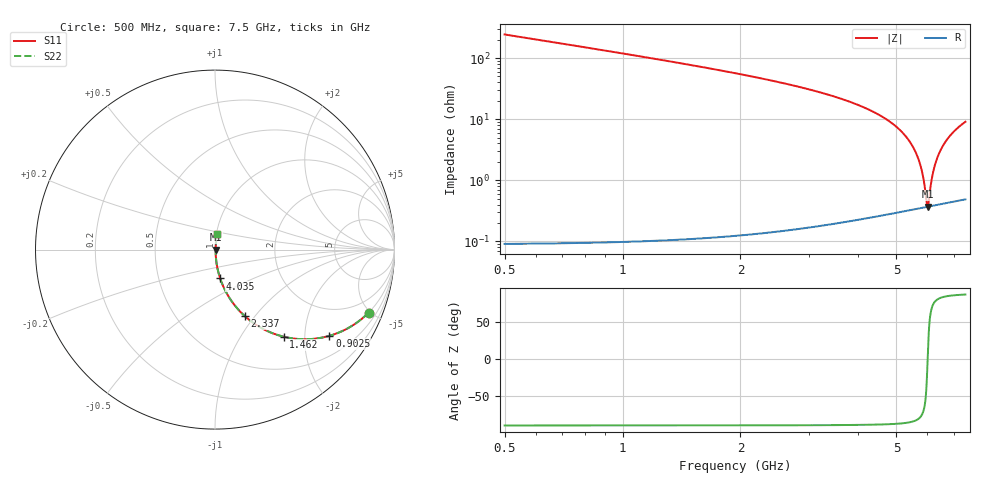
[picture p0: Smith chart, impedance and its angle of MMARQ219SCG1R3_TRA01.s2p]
! MMARQ219SCG1R3_TRA01  S-PARAMETER MODEL  ( General Type )
! Model Generated by TAIYO YUDEN Corporation (http://www.ty-top.com)
! Version 1.0
! TAIYO YUDEN Control No. 180601
! Copyright(c) 2018 TAIYO YUDEN CO.,LTD. All Rights Reserved.
! Product Description (link to TY-COMPAS)
! https://ds.yuden.co.jp/TYCOMPAS/or/detail?pn=MMARQ219SCG1R3BTRA01&u=M
! Products Name : Multilayer Ceramic Capacitors
! Characteristics :
!  Capacitance : 1.3 pF , Rated Voltage : 250V , TCC : CG / C0G
!  Case Size : 2.0 x 1.25 / 0.079 x 0.049 [mm/inch] , Thickness : 0.85 / 0.033 [mm/inch]
!  (Conditions: Temperature = 25 degC , DC Bias Current/Voltage = 0A / 0V)
! External Node Assignments :
!  1  o---| |---o  2
! GND o---------o GND
! Frequency Range : 500MHz  -  7500MHz  [ 401 STEP ]
# MHz S RI R 50
! Freq[MHz].  S11 Real  S11 Imag  S21 Real  S21 Imag  S12 Real  S12 Imag  S22 Real  S22 Imag
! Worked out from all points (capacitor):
!   401 points, 500 MHz to 7.5 GHz, reference 50 ohm
!   read as one part in series: C = 1.3 pF near 535 MHz
!   lowest |Z| = 370 mohm at 6.013 GHz (marker M1)
!   series resonance near 6.008 GHz, so ESL is about 540 pH
!   S11 on the Smith chart (normalised r, x): 500 MHz: 1.00, -4.86; 902.5 MHz: 1.00, -2.65; 1.462 GHz: 1.00, -1.57; 2.337 GHz: 1.00, -0.89; 4.035 GHz: 1.00, -0.33; 7.5 GHz: 1.01, +0.18
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500  0.8553 -0.3516  0.1447 0.3516  0.1447 0.3516  0.8553 -0.3516
902.5  0.6373 -0.4804  0.3627 0.4804  0.3627 0.4804  0.6373 -0.4804
1462.5  0.3828 -0.4854  0.6172 0.4854  0.6172 0.4854  0.3828 -0.4854
1672.5  0.3133 -0.463  0.6867 0.463  0.6867 0.463  0.3133 -0.463
2337.5  0.1655 -0.3701  0.8345 0.3701  0.8345 0.3701  0.1655 -0.3701
2845  0.1012 -0.2992  0.8988 0.2992  0.8988 0.2992  0.1012 -0.2992
4000  0.0302 -0.1645  0.9698 0.1645  0.9698 0.1645  0.0302 -0.1645
4035  0.029 -0.161  0.971 0.161  0.971 0.161  0.029 -0.161
4682.5  0.013 -0.1007  0.987 0.1007  0.987 0.1007  0.013 -0.1007
5172.5  0.00673 -0.0604  0.9933 0.0604  0.9933 0.0604  0.00673 -0.0604
5470  0.00471 -0.0378  0.9953 0.0378  0.9953 0.0378  0.00471 -0.0378
5697.5  0.0039 -0.0214  0.9961 0.0214  0.9961 0.0214  0.0039 -0.0214
5837.5  0.00368 -0.0116  0.9963 0.0116  0.9963 0.0116  0.00368 -0.0116
5977.5  0.00366 -0.00205  0.9963 0.00205  0.9963 0.00205  0.00366 -0.00205
6012.5  0.00368 0.000299  0.9963 -0.000299  0.9963 -0.000299  0.00368 0.000299
6047.5  0.00371 0.00263  0.9963 -0.00263  0.9963 -0.00263  0.00371 0.00263
6117.5  0.00381 0.00727  0.9962 -0.00727  0.9962 -0.00727  0.00381 0.00727
6187.5  0.00395 0.0118  0.996 -0.0118  0.996 -0.0118  0.00395 0.0118
6345  0.00442 0.0219  0.9956 -0.0219  0.9956 -0.0219  0.00442 0.0219
6537.5  0.00524 0.0339  0.9948 -0.0339  0.9948 -0.0339  0.00524 0.0339
6782.5  0.00667 0.0487  0.9933 -0.0487  0.9933 -0.0487  0.00667 0.0487
7500  0.0129 0.0889  0.9871 -0.0889  0.9871 -0.0889  0.0129 0.0889
